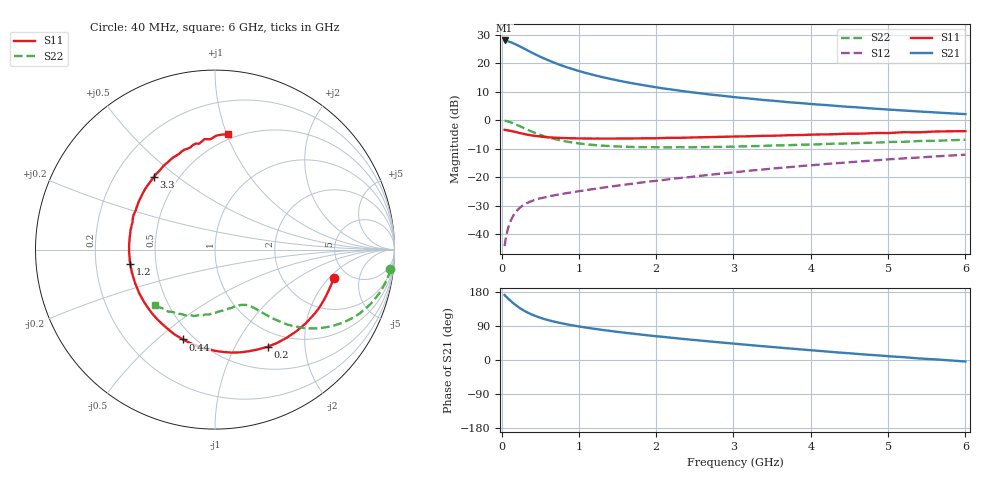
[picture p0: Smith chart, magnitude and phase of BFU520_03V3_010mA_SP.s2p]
! Filename:  P:\Prog\Test\Noise\ATS_data\Testdata_Net\03 Spar\BFU520_APG2013_37_A05_03p3V_010mA_SP_CM01_D.s2p
! Date/Time: Fri 26/Apr/2013 13:00:07
! BFU520_APG2013_37_A05_03p3V_1to20mA_SP_CM01_Bias6_R.s2p
! MDIF S-parameter v. bias file
! BFU520_APG2013_37_A05_03p3V_1to20mA_SP_CM01
! Date/time Tue Apr 23 14:11:50 2013
! VAR V_out= 3.3000
! VAR I_out= 9.9950
! VAR V_in= 0.8451
! VAR I_in= 0.1172
! Device data file deembeded for feedlines and parallel
! Original file: \03 Spar\BFU520_APG2013_37_A05_03p3V_010mA_SP_CM01_R.s2p
! Feed-files: PR047V01_250413_Feed1.s2p, PR047V01_250413_Feed2.s2p
! Parallel-file: PR047V01_250413_Par.s2p
# MHz S MA R 50
!  Freq-MHz  S11-mag  S11-arg  S21-mag  S21-arg  S12-mag  S12-arg  S22-mag  S22-arg
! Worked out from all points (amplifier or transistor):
!   98 points, 40 MHz to 6 GHz, reference 50 ohm
!   highest |S21| = 28.0 dB at 40 MHz (marker M1)
!   |S21| within 3 dB of that: start of sweep to 303.5 MHz
!   unconditionally stable (mu >= 1): 1.698 GHz to 3.856 GHz
!   at 300 MHz: K = 0.32, MSG = 27.3 dB, |S12| = -29.5 dB
!   at 1.6 GHz: K = 0.98, MSG = 18.0 dB, |S12| = -22.6 dB
!   at 6 GHz: K = 0.85, MSG = 7.1 dB, |S12| = -12.1 dB
!   S11 on the Smith chart (normalised r, x): 40 MHz: 3.84, -2.25; 200 MHz: 0.78, -1.36; 440 MHz: 0.44, -0.61; 1.2 GHz: 0.35, -0.08; 3.3 GHz: 0.37, +0.42; 6 GHz: 0.46, +1.01
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40  0.6789 -13.5  25.14 171.4  0.006204 83.4  0.9817 -6.5
50  0.6766 -16.8  25.13 168.8  0.007709 82.2  0.9791 -8.1
60  0.6728 -19.9  24.66 167.2  0.009217 80.8  0.9724 -9.8
120  0.6513 -39.1  23.43 155.6  0.0174 72.6  0.9213 -18.8
160  0.6332 -50.8  22.18 148.7  0.02211 67.6  0.8788 -24.1
200  0.6152 -61.6  20.92 142.4  0.02611 63.6  0.8312 -28.7
240  0.5965 -71.8  19.71 136.7  0.0295 60.2  0.7855 -32.6
300  0.5728 -85.1  17.9 129.2  0.03365 56.2  0.7203 -37.5
380  0.5465 -100.2  15.69 121.1  0.03788 52.4  0.6445 -42.4
440  0.5316 -109.6  14.29 116.0  0.04052 50.6  0.5978 -45.0
550  0.5098 -124.3  12.17 108.3  0.04421 48.5  0.5277 -48.5
700  0.495 -138.9  10.02 100.3  0.04881 47.6  0.4653 -51.7
850  0.4871 -150.4  8.476 94.0  0.05296 47.7  0.4224 -54.0
1050  0.4801 -162.7  7.006 86.9  0.05839 48.6  0.3863 -56.7
1200  0.4786 -170.1  6.189 82.3  0.06259 49.4  0.3685 -58.5
1600  0.4791 173.8  4.707 71.8  0.07442 51.1  0.3439 -63.7
2050  0.4871 160.5  3.697 61.8  0.08827 52.3  0.3362 -70.5
3100  0.5217 134.1  2.481 41.5  0.1262 52.0  0.3485 -87.8
3300  0.5298 129.8  2.336 37.8  0.1342 51.3  0.3534 -91.2
4100  0.5643 114.1  1.887 24.2  0.1668 47.7  0.3787 -105.0
5200  0.6186 95.4  1.486 7.5  0.2146 40.6  0.4194 -124.0
6000  0.6454 83.8  1.284 -3.9  0.2493 34.2  0.4561 -137.5
